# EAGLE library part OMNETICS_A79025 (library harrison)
Omnetics A79025 36-pin connector
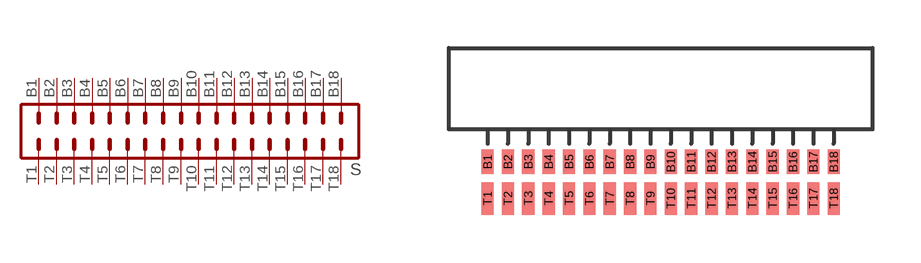
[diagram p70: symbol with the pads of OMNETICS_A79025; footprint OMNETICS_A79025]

Designator prefix S

## OMNETICS_A79025  [OMNETICS_A79025]
B1  B1  pas
B2  B2  pas
B3  B3  pas
B4  B4  pas
B5  B5  pas
B6  B6  pas
B7  B7  pas
B8  B8  pas
B9  B9  pas
B10  B10  pas
B11  B11  pas
B12  B12  pas
B13  B13  pas
B14  B14  pas
B15  B15  pas
B16  B16  pas
B17  B17  pas
B18  B18  pas
T1  T1  pas
T2  T2  pas
T3  T3  pas
T4  T4  pas
T5  T5  pas
T6  T6  pas
T7  T7  pas
T8  T8  pas
T9  T9  pas
T10  T10  pas
T11  T11  pas
T12  T12  pas
T13  T13  pas
T14  T14  pas
T15  T15  pas
T16  T16  pas
T17  T17  pas
T18  T18  pas

## Footprint OMNETICS_A79025 (pad centres in mm)
smd 0.381 x 0.762: B1 -5.397,-1.016; B2 -4.763,-1.016; B3 -4.128,-1.016; B4 -3.493,-1.016; B5 -2.857,-1.016; B6 -2.223,-1.016; B7 -1.587,-1.016; B8 -0.953,-1.016; B9 -0.318,-1.016; B10 0.318,-1.016; B11 0.953,-1.016; B12 1.587,-1.016; B13 2.223,-1.016; B14 2.857,-1.016; B15 3.493,-1.016; B16 4.128,-1.016; B17 4.763,-1.016; B18 5.397,-1.016
smd 0.381 x 1.016: T1 -5.397,-2.159; T2 -4.763,-2.159; T3 -4.128,-2.159; T4 -3.493,-2.159; T5 -2.857,-2.159; T6 -2.223,-2.159; T7 -1.587,-2.159; T8 -0.953,-2.159; T9 -0.318,-2.159; T10 0.318,-2.159; T11 0.953,-2.159; T12 1.587,-2.159; T13 2.223,-2.159; T14 2.857,-2.159; T15 3.493,-2.159; T16 4.128,-2.159; T17 4.763,-2.159; T18 5.397,-2.159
